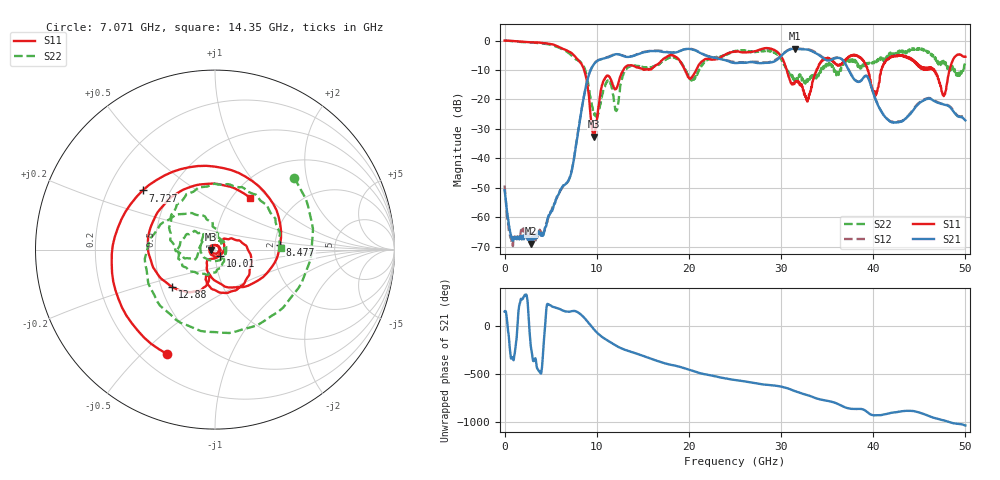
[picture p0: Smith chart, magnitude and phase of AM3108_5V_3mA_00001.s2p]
# Hz S DB R 50.0
!freq dBS11 angS11 dBS21 angS21 dBS12 angS12 dBS22 angS22
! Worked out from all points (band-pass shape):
!   1601 points, 10 MHz to 50 GHz, reference 50 ohm
!   highest |S21| = -2.78 dB at 31.53 GHz (marker M1); lowest = -69.0 dB at 2.853 GHz (marker M2)
!   |S21| within 3 dB of the highest: 11.16 GHz to 22.69 GHz (11.53 GHz wide, 68.1 % of centre); 29.83 GHz to 34.47 GHz (4.636 GHz wide, 14.4 % of centre)
!   lowest |S11| = -32.7 dB at 9.664 GHz (marker M3), VSWR 1.05, Z = 47.7 - j0.107 ohm
!   |S11| at or under -10 dB: 8.638 GHz to 12.88 GHz (4.24 GHz wide, 39.4 % of centre); 30.63 GHz to 33.85 GHz (3.219 GHz wide, 9.99 % of centre); 46.63 GHz to 48.29 GHz (1.659 GHz wide, 3.49 % of centre)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
!   |S22| runs from -26.4 to 0.0 dB; largest |S21 - S12| = 0.024
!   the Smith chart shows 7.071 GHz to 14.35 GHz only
!   S11 on the Smith chart (normalised r, x): 7.071 GHz: 0.30, -0.60; 7.727 GHz: 0.35, +0.32; 8.477 GHz: 2.13, +0.13; 10.01 GHz: 1.05, -0.07; 12.88 GHz: 0.57, -0.26; 14.35 GHz: 1.20, +0.79
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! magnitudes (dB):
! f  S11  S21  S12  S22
! 10 MHz  0.0  -50.8  -49.2  0.0
! 728.6 MHz  -0.1  -66.2  -67.0  -0.2
! 2.853 GHz  -0.6  -69.0  -65.7  -0.7
! 7.071 GHz  -3.9  -46.6  -46.6  -4.5
! 7.727 GHz  -5.7  -36.2  -36.0  -6.3
! 8.352 GHz  -8.0  -23.6  -23.5  -7.6
! 8.477 GHz  -8.8  -21.3  -21.3  -8.1
! 9.664 GHz  -32.7  -8.2  -8.1  -24.0
! 10.01 GHz  -27.2  -7.0  -7.0  -25.8
! 10.82 GHz  -13.2  -6.0  -6.0  -16.3
! 12.13 GHz  -16.3  -4.6  -4.6  -23.9
! 12.88 GHz  -10.0  -5.3  -5.1  -11.6
! 14.35 GHz  -9.2  -4.8  -4.7  -8.7
! 16.69 GHz  -7.9  -3.6  -3.4  -8.3
! 25 GHz  -3.7  -7.7  -7.3  -3.7
! 31.53 GHz  -14.1  -2.8  -2.6  -13.8
! 33.35 GHz  -15.6  -3.6  -3.4  -12.7
! 38 GHz  -4.8  -13.4  -13.3  -6.6
! 40.22 GHz  -18.8  -19.8  -19.6  -7.6
! 41.69 GHz  -6.1  -27.1  -27.0  -5.2
! 47.66 GHz  -18.9  -21.7  -21.6  -7.7
! 50 GHz  -5.5  -27.1  -26.5  -6.9
